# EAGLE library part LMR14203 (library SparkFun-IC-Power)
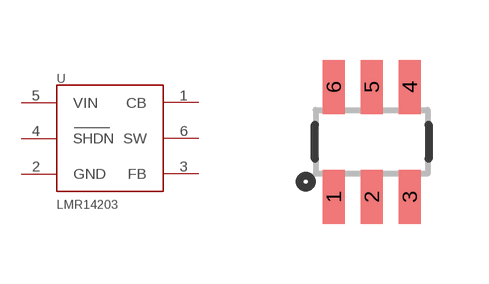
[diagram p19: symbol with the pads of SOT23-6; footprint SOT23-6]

Designator prefix -

## LMR14203 (PROD_ID: IC-13918)  [SOT23-6]
1  CB  in
2  GND  pwr
3  FB  in
4  SHDN  in
5  VIN  pwr
6  SW  pwr

## Footprint SOT23-6 (pad centres in mm)
smd 0.55 x 1.35: 1 -0.95,-1.375; 2 0,-1.375; 3 0.95,-1.375; 4 0.95,1.375; 5 0,1.375; 6 -0.95,1.375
